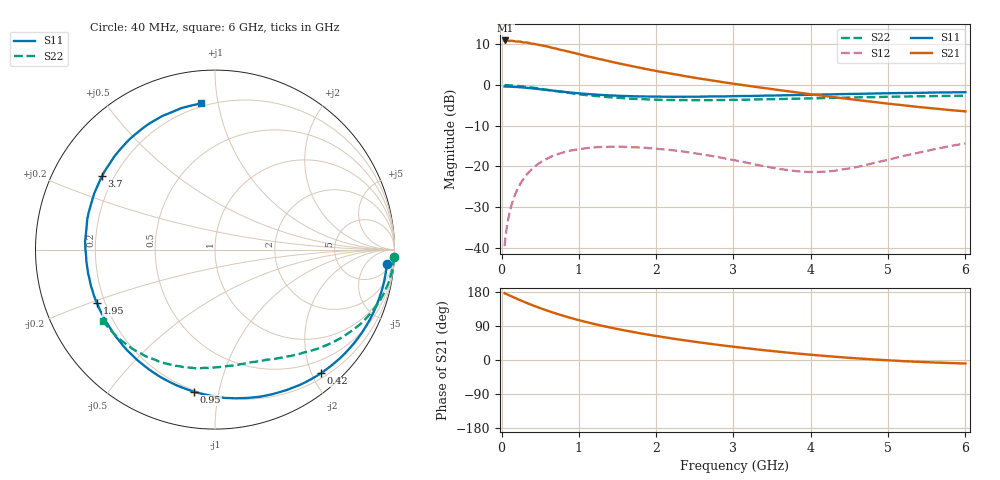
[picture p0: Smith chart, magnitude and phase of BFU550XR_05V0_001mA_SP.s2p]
! Filename:  P:\Prog\Test\Noise\ATS_data\Testdata_Net\03 Spar\BFU550XR_APG2013_45_C05_05p0V_001mA_SP_CM01_D.s2p
! Date/Time: Tue 06/Aug/2013 14:38:15
! BFU550XR_APG2013_45_C05_05p0V_1to35mA_SP_CM01_Bias1_R.s2p
! MDIF S-parameter v. bias file
! BFU550XR_APG2013_45_C05_05p0V_1to35mA_SP_CM01
! Date/time Fri Aug 02 14:46:46 2013
! bias mode 1
! bias variable = I_out
! VAR bias_var= 1
! VAR V_out= 5.0000
! VAR I_out= 0.9950
! VAR V_in= 0.7767
! VAR I_in= 0.0107
! Device data file deembeded for feedlines and parallel
! Original file: \03 Spar\BFU550XR_APG2013_45_C05_05p0V_001mA_SP_CM01_R.s2p
! Feed-files: PR006V01_02082013_Feed1.s2p, PR006V01_02082013_Feed2.s2p
! Parallel-file: PR006V01_02082013_Par.s2p
# MHz S MA R 50
!  Freq-MHz  S11-mag  S11-arg  S21-mag  S21-arg  S12-mag  S12-arg  S22-mag  S22-arg
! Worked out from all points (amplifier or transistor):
!   98 points, 40 MHz to 6 GHz, reference 50 ohm
!   highest |S21| = 11.0 dB at 50 MHz (marker M1)
!   |S21| within 3 dB of that: start of sweep to 924.4 MHz
!   unconditionally stable (mu >= 1): 3.431 GHz to 4.835 GHz
!   at 300 MHz: K = 0.09, MSG = 16.6 dB, |S12| = -22.7 dB
!   at 1.6 GHz: K = 0.38, MSG = 10.1 dB, |S12| = -15.2 dB
!   at 6 GHz: K = 0.79, MSG = 3.9 dB, |S12| = -14.3 dB
!   S11 on the Smith chart (normalised r, x): 40 MHz: 9, -19; 420 MHz: 0.28, -2.14; 950 MHz: 0.19, -0.84; 1.95 GHz: 0.17, -0.21; 3.7 GHz: 0.15, +0.29; 6 GHz: 0.18, +0.89
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40  0.9612 -4.9  3.53 176.4  0.01045 86.8  0.9981 -2.3
50  0.9603 -6.1  3.54 174.9  0.0131 86.1  0.9988 -3.0
100  0.9578 -12.3  3.494 170.6  0.02595 82.0  0.9936 -6.2
180  0.9495 -21.9  3.451 163.3  0.04607 75.7  0.9834 -11.1
240  0.9406 -29.1  3.429 158.0  0.06021 71.3  0.9717 -14.7
320  0.9266 -38.5  3.346 151.1  0.0779 65.5  0.9525 -19.2
420  0.9066 -49.5  3.212 143.0  0.0977 58.8  0.9254 -24.3
600  0.8669 -68.2  2.977 129.7  0.1261 47.8  0.8723 -32.8
800  0.8281 -86.3  2.676 116.7  0.1487 37.5  0.8189 -40.5
950  0.8009 -98.5  2.473 107.9  0.1598 30.6  0.7825 -45.6
1050  0.7857 -105.9  2.338 102.5  0.1651 26.7  0.7615 -48.6
1250  0.7614 -119.3  2.108 92.7  0.1731 19.5  0.7313 -53.9
1500  0.7406 -133.8  1.865 81.8  0.1749 11.8  0.6983 -60.3
1700  0.729 -144.1  1.702 74.0  0.1715 6.7  0.6763 -65.1
1950  0.7213 -155.5  1.523 65.1  0.167 1.1  0.6644 -70.3
2050  0.7214 -159.7  1.462 61.9  0.1632 -0.7  0.6586 -72.5
2500  0.7188 -176.8  1.231 48.1  0.1453 -7.4  0.6533 -81.6
3100  0.7334 163.8  1.009 32.6  0.1148 -8.9  0.6604 -93.5
3700  0.7509 147.0  0.8417 19.5  0.09018 1.4  0.6779 -105.1
4100  0.7646 136.8  0.7514 12.1  0.08551 16.0  0.6896 -112.7
5200  0.8001 111.6  0.5645 -3.0  0.1345 41.7  0.7225 -133.1
6000  0.818 95.5  0.4751 -9.2  0.1918 40.6  0.7409 -147.3
